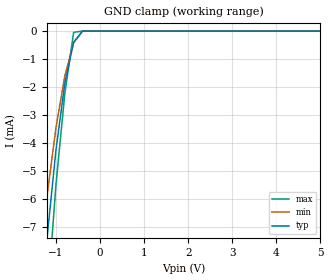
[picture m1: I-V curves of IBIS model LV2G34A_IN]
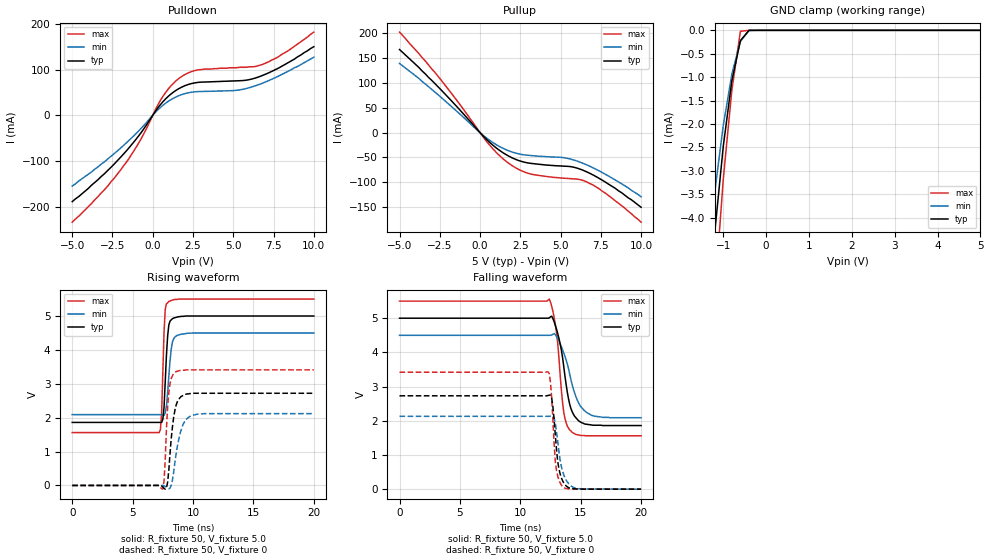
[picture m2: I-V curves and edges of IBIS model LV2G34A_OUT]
|/_/_/_/_/_/_/_/_/_/_/_/_/_/_/_/_/_/_/_/_/_/_/_/_/_/_/_/_/_/_/_/_/_/_/_/_/_/
|   Renesas Electronics Corp.
|   Multi Purpose Semiconductor Digital IC Design Group
|   IBIS Model of HD74LV2G34A
|   5.0V Triple Noninverters,  SSOP-8(8pin) Package
|   History
|   V1.0   April   1, 2003   : First release.
|/_/_/_/_/_/_/_/_/_/_/_/_/_/_/_/_/_/_/_/_/_/_/_/_/_/_/_/_/_/_/_/_/_/_/_/_/_/
[IBIS Ver]   2.1
[Comment Char]  |_char
[File name]   l2g34s5.ibs
[File Rev]   1.1
[Date]   April 1, 2003
[Source]   Data created from SPICE simulations at
|   Renesas Electronics Corp.
[Notes]   RLC value of the Package is determined by assuming typical
|   conditions.
[Disclaimer]   This information is for modeling purposes only, and is not
|   guaranteed.
[Copyright]   Copyright 2003, Renesas Electronics Corp.,
|   All Rights Reserved.
|   Component  HD74LV2G34A
[Component]   HD74LV2G34A
[Manufacturer]  Renesas Electronics Corp.
[Package]
|   typ   min   max
R_pkg   0.099   0.095   0.102
L_pkg   1.740nH   1.680nH   1.790nH
C_pkg   0.140pF   0.140pF   0.150pF
[Pin]   signal_name   model_name   R_pin   L_pin   C_pin
1   1A   LV2G34A_IN   0.102   1.780nH   0.140pF
2   3Y   LV2G34A_OUT   0.097   1.710nH   0.150pF
3   2A   LV2G34A_IN   0.095   1.680nH   0.150pF
4   GND   GND   0.102   1.790nH   0.140pF
5   2Y   LV2G34A_OUT   0.101   1.790nH   0.140pF
6   3A   LV2G34A_IN   0.097   1.710nH   0.150pF
7   1Y   LV2G34A_OUT   0.097   1.710nH   0.150pF
8   VCC   POWER   0.102   1.790nH   0.140pF
| Models and submodels in the file (2): LV2G34A_IN (Input), LV2G34A_OUT (Output)
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|   Model  LV2G34A_IN
[Model]   LV2G34A_IN
Model_type  Input
Vinl = 1.50V
Vinh = 3.50V
| variable   typ   min   max
C_comp   2.35pF   2.25pF   2.45pF
| variable   typ   min   max
[Temperature range]   25   85   -40
| variable   typ   min   max
[Voltage range]   5.0V   4.5V   5.5V
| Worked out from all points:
|   GND clamp passes 1 mA (typ) near -0.68 V on its own axis
[GND Clamp]
|   Voltage   I(typ)   I(min)   I(max)
-5V       -128mA     -106mA     -157mA
-1.4V     -11mA      -8.74mA    -14.7mA
-1.2V     -7.33mA    -5.84mA    -9.68mA
-1V       -4.23mA    -3.44mA    -5.46mA
-800mV    -1.86mA    -1.6mA     -2.23mA
-600mV    -396uA     -418uA     -43uA
-400mV    -474nA     -10.9uA    -2.94nA
5V        10.1pA     35.9pA     10pA
|   Model  LV2G34A_OUT
[Model]   LV2G34A_OUT
Model_type  Output
Polarity   Inverting
Vmeas = 2.50V
| variable   typ   min   max
C_comp   8.35pF   8.25pF   8.45pF
| variable   typ   min   max
[Temperature range]   25   85   -40
| variable   typ   min   max
[Voltage range]   5.0V   4.5V   5.5V
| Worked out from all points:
|   slope of the pulldown table from 0 to 0.75 V, typ, clamps not added: 22 ohm
|   slope of the pullup table from 0 to 0.75 V, typ, clamps not added: 31.4 ohm
|   GND clamp passes 1 mA (typ) near -0.78 V on its own axis
|   rising waveform, R_fixture 50, V_fixture 5.0: 20-80 % time 267ps typ, 340ps min, 211ps max; typ from 1.86 V to 5 V
|   rising waveform, R_fixture 50, V_fixture 0: 20-80 % time 463ps typ, 662ps min, 306ps max; typ from 0 V to 2.72 V
|   falling waveform, R_fixture 50, V_fixture 5.0: 20-80 % time 865ps typ, 1.2ns min, 620ps max; typ from 5 V to 1.86 V
|   falling waveform, R_fixture 50, V_fixture 0: 20-80 % time 472ps typ, 606ps min, 364ps max; typ from 2.73 V to 0 V
[Pullup]
|   Voltage   I(typ)   I(min)   I(max)
-5V       167mA      139mA      202mA
-2.4V     85.2mA     70.3mA     105mA
200mV     -6.98mA    -5.55mA    -8.94mA
1V        -30.6mA    -24.1mA    -39.5mA
1.6V      -43.9mA    -34.1mA    -57.2mA
2.4V      -56.1mA    -42.7mA    -74mA
3.2V      -62mA      -46.2mA    -83.6mA
5.2V      -67.4mA    -50.4mA    -91.6mA
5.8V      -69.4mA    -54.8mA    -92.9mA
6.6V      -78.5mA    -64.5mA    -98.7mA
7.8V      -99.8mA    -84mA      -122mA
10V       -150mA     -129mA     -180mA
[Pulldown]
|   Voltage   I(typ)   I(min)   I(max)
-5V       -189mA     -155mA     -234mA
-3V       -128mA     -102mA     -163mA
-1.6V     -76.4mA    -59.1mA    -101mA
-800mV    -41.6mA    -31.5mA    -56.3mA
600mV     28.4mA     20.9mA     39.7mA
1V        42.6mA     31.4mA     59.1mA
1.6V      57.9mA     42.5mA     79.9mA
2.8V      71.9mA     51.8mA     99.3mA
5.2V      75.3mA     54.5mA     104mA
6.8V      86.9mA     70mA       111mA
8.4V      115mA      96.1mA     141mA
10V       150mA      127mA      182mA
[GND Clamp]
|   Voltage   I(typ)   I(min)   I(max)
-5V       -76.6mA    -64mA      -93.9mA
-1.4V     -6.55mA    -5.21mA    -8.67mA
-1.2V     -4.33mA    -3.47mA    -5.69mA
-1V       -2.48mA    -2.03mA    -3.18mA
-800mV    -1.08mA    -936uA     -1.28mA
-600mV    -219uA     -237uA     -20.5uA
-400mV    -248nA     -6.13uA    -1.4nA
5V        5.14pA     37.3pA     5pA
[Ramp]
| variable   typ   min   max
dV/dt_r   1.636/465.5p   1.276/663.3p   2.049/306.9p
dV/dt_f   1.882/862.6p   1.447/1.200n   2.363/618.8p
R_load = 50ohms
[Rising Waveform]
R_fixture = 50
V_fixture = 5.0
V_fixture_min = 4.5
V_fixture_max = 5.5
C_fixture = 0p
|   Time   V(typ)   V(min)   V(max)
0s        1.86V      2.09V      1.56V
7.2ns     1.86V      2.09V      1.56V
7.4ns     1.86V      2.08V      2.14V
7.6ns     2.3V       2.07V      4.52V
7.7ns     3.07V      2.14V      5.2V
7.9ns     4.42V      2.75V      5.39V
8ns       4.74V      3.25V      5.43V
8.3ns     4.92V      4.24V      5.47V
8.7ns     4.97V      4.43V      5.49V
20ns      5V         4.5V       5.5V
[Rising Waveform]
R_fixture = 50
V_fixture = 0
C_fixture = 0p
|   Time   V(typ)   V(min)   V(max)
0s        402pV      815nV      126pV
7.5ns     -46.3mV    2.17mV     -106mV
7.6ns     -84.2mV    -10.8mV    125mV
7.8ns     -74.4mV    -57.3mV    1.68V
8ns       472mV      -98.5mV    2.76V
8.3ns     1.74V      164mV      3.24V
8.6ns     2.37V      929mV      3.36V
9.1ns     2.64V      1.73V      3.4V
9.8ns     2.71V      2.05V      3.41V
20ns      2.72V      2.12V      3.41V
[Falling Waveform]
R_fixture = 50
V_fixture = 5.0
V_fixture_min = 4.5
V_fixture_max = 5.5
C_fixture = 0p
|   Time   V(typ)   V(min)   V(max)
0s        5V         4.5V       5.5V
12.4ns    5.01V      4.5V       5.56V
12.6ns    5.06V      4.51V      5.35V
12.9ns    4.79V      4.52V      4.82V
13.2ns    4.41V      4.33V      3.83V
13.6ns    3.58V      3.98V      2.24V
14ns      2.63V      3.51V      1.78V
14.7ns    2.05V      2.62V      1.59V
15.5ns    1.9V       2.24V      1.56V
20ns      1.86V      2.09V      1.56V
[Falling Waveform]
R_fixture = 50
V_fixture = 0
C_fixture = 0p
|   Time   V(typ)   V(min)   V(max)
0s        2.73V      2.13V      3.42V
12.3ns    2.74V      2.13V      3.43V
12.5ns    2.75V      2.14V      3.12V
12.7ns    2.41V      2.14V      2.01V
12.9ns    1.58V      1.93V      810mV
13.1ns    805mV      1.39V      381mV
13.4ns    332mV      664mV      120mV
13.9ns    65.5mV     207mV      12.9mV
14.6ns    7.61mV     28.1mV     1.53mV
20ns      -26.1uV    -57.9uV    -7.77uV
